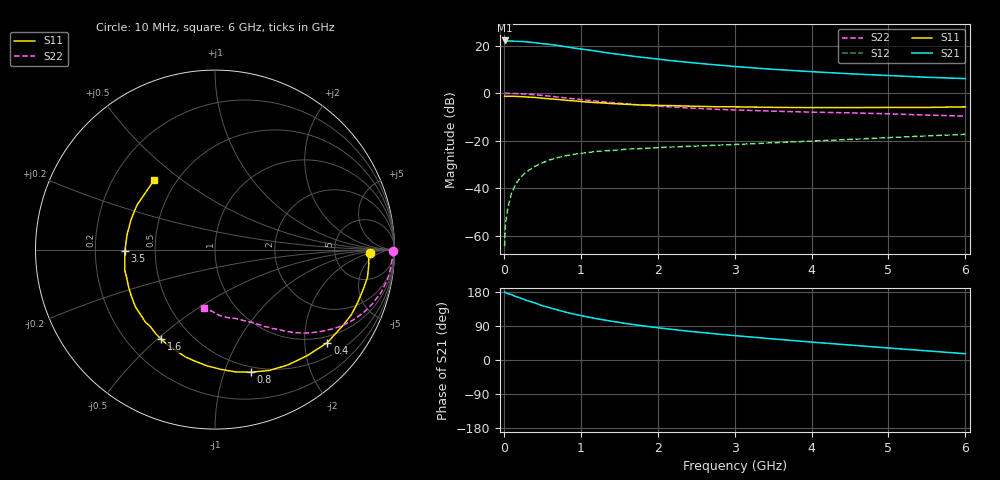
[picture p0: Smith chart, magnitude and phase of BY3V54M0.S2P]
! SIEMENS Small Signal Semiconductors
! BFY420
! Si NPN RF SIEGET Grounded Emitter Transistor in MICRO-X
! VCE = 3.5 V  IC = 4 mA
! Common Emitter S-Parameters:  October  1996
# GHz  S  MA  R  50
!  f  S11  S21  S12  S22
! GHz  MAG  ANG  MAG  ANG  MAG  ANG  MAG  ANG
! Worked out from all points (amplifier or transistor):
!   36 points, 10 MHz to 6 GHz, reference 50 ohm
!   highest |S21| = 22.2 dB at 10 MHz (marker M1)
!   |S21| within 3 dB of that: start of sweep to 874.4 MHz
!   unconditionally stable (mu >= 1): 3.366 GHz to end of sweep
!   at 250 MHz: K = 0.12, MSG = 28.1 dB, |S12| = -34.4 dB
!   at 1.4 GHz: K = 0.46, MSG = 20.4 dB, |S12| = -24.1 dB
!   at 6 GHz: K = 1.16, MAG = 9.3 dB, |S12| = -17.3 dB
!   S11 on the Smith chart (normalised r, x): 10 MHz: 13, -2; 400 MHz: 0.83, -2.54; 800 MHz: 0.45, -1.24; 1.6 GHz: 0.34, -0.51; 3.5 GHz: 0.33, -0.01; 6 GHz: 0.38, +0.40
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0.01  0.8634 -1.2  12.88 179.9  0.0006 54.4  0.9906 -0.4
0.02  0.8558 -2.2  12.78 177.8  0.0017 65.8  0.9887 -0.9
0.05  0.8609 -5.2  12.55 175.3  0.0037 84.1  0.9903 -2.4
0.1  0.8634 -10.3  12.5 172.4  0.0078 82.2  0.9851 -5.0
0.15  0.8546 -15.3  12.39 167.7  0.0118 78.5  0.9811 -7.5
0.2  0.8481 -20.4  12.3 164.8  0.0155 77.1  0.9748 -9.9
0.25  0.8418 -25.5  12.23 160.7  0.019 74.1  0.9643 -12.2
0.4  0.8128 -39.6  11.58 150.8  0.0286 68.3  0.9272 -19.1
0.5  0.7831 -48.9  11.02 143.4  0.034 64.5  0.8973 -23.2
0.6  0.7603 -57.7  10.63 137.7  0.0396 60.7  0.8638 -27.0
0.8  0.7123 -73.5  9.526 126.5  0.048 52.9  0.7965 -33.5
0.9  0.6915 -80.3  8.984 121.6  0.0512 50.7  0.7651 -36.0
1.1  0.6484 -94.2  8.135 113.2  0.0565 46.2  0.707 -40.9
1.4  0.6041 -110.7  6.857 102.3  0.0621 41.4  0.6357 -46.6
1.6  0.5821 -121.0  6.232 95.8  0.0663 39.1  0.5937 -49.7
1.9  0.5601 -133.9  5.464 87.8  0.07 36.5  0.5465 -53.7
2.2  0.5462 -144.3  4.793 80.5  0.0737 34.9  0.5106 -57.1
2.8  0.5165 -162.0  3.893 68.1  0.0807 33.1  0.4547 -63.1
3.5  0.5023 -179.1  3.177 55.6  0.0903 31.9  0.4181 -69.5
4.5  0.4969 160.2  2.56 39.5  0.1062 29.2  0.3854 -79.5
5.5  0.5008 140.2  2.163 24.2  0.1261 25.4  0.3452 -92.5
6  0.5153 131.1  2.028 16.6  0.1359 22.6  0.3282 -100.3
